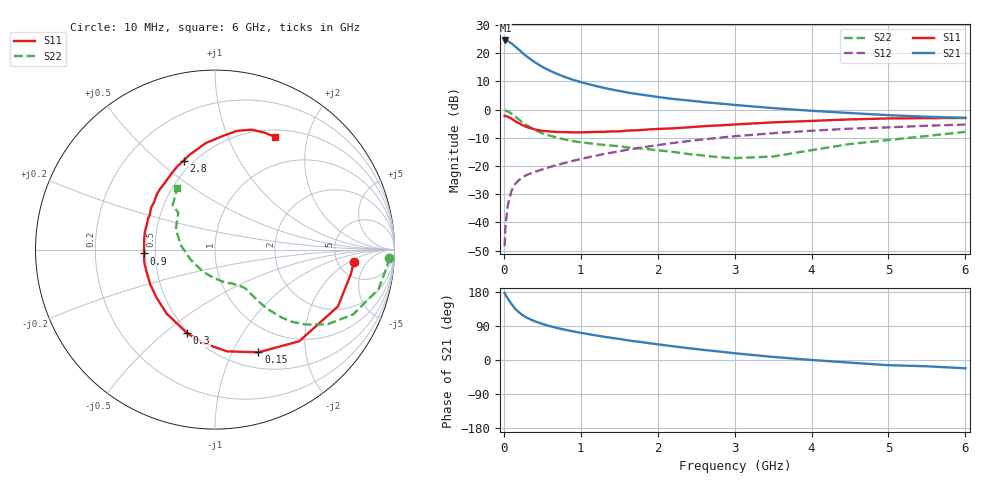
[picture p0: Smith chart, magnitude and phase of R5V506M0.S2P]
! SIEMENS Small Signal Semiconductors
! BFR183
! Si NPN RF Bipolar Junction Transistor in SOT23
! VCE = 0.5 V  IC = 6 mA
! Common Emitter S-Parameters:  May  1996
# GHz  S  MA  R  50
!  f  S11  S21  S12  S22
! GHz  MAG  ANG  MAG  ANG  MAG  ANG  MAG  ANG
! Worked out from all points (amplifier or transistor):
!   36 points, 10 MHz to 6 GHz, reference 50 ohm
!   highest |S21| = 24.5 dB at 20 MHz (marker M1)
!   |S21| within 3 dB of that: start of sweep to 184.2 MHz
!   unconditionally stable (mu >= 1): 830 MHz to 3.439 GHz
!   at 250 MHz: K = 0.49, MSG = 21.9 dB, |S12| = -23.9 dB
!   at 1.4 GHz: K = 1.10, MAG = 9.2 dB, |S12| = -15.2 dB
!   at 6 GHz: K = 0.98, MSG = 1.2 dB, |S12| = -5.3 dB
!   S11 on the Smith chart (normalised r, x): 10 MHz: 7.09, -2.47; 150 MHz: 0.68, -1.27; 300 MHz: 0.49, -0.60; 900 MHz: 0.43, -0.02; 2.8 GHz: 0.45, +0.61; 6 GHz: 0.59, +1.50
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0.01  0.7768 -5.1  16.82 176.8  0.0038 87.6  0.9727 -2.7
0.02  0.7691 -10.1  16.87 172.8  0.0082 86.9  0.9633 -5.5
0.05  0.7547 -24.8  16.56 162.7  0.0198 77.1  0.9375 -13.6
0.1  0.6935 -47.4  14.92 147.7  0.0365 66.9  0.8506 -25.1
0.15  0.6212 -67.1  13.12 134.6  0.0486 60.5  0.7522 -33.6
0.2  0.5708 -83.3  11.44 125.1  0.0571 55.9  0.6601 -39.3
0.25  0.5264 -96.3  9.904 117.6  0.064 52.8  0.5869 -43.2
0.3  0.4914 -108.3  8.724 111.4  0.0698 51.6  0.5286 -45.6
0.4  0.4467 -127.2  6.99 102.3  0.0788 50.5  0.4384 -48.6
0.5  0.4219 -140.4  5.735 95.2  0.0873 50.5  0.3801 -49.9
0.6  0.41 -151.5  4.899 89.3  0.0963 50.9  0.3456 -50.4
0.7  0.4015 -161.3  4.271 84.1  0.1052 51.7  0.3174 -51.0
0.9  0.3962 -176.9  3.383 75.5  0.1241 52.9  0.2764 -52.0
1.1  0.3996 170.6  2.834 68.3  0.1433 53.2  0.2548 -54.3
1.3  0.404 160.3  2.437 61.5  0.1635 52.6  0.2372 -56.7
1.6  0.4255 146.8  2.023 52.3  0.194 51.6  0.2155 -62.2
2.2  0.4665 126.4  1.549 36.2  0.2568 46.8  0.1784 -79.0
2.8  0.5254 109.4  1.286 22.4  0.3182 40.2  0.1434 -108.1
3.5  0.5954 95.0  1.066 8.1  0.3823 30.8  0.1477 -158.6
4.5  0.6724 79.6  0.871 -7.0  0.461 17.9  0.2458 152.5
5.5  0.7074 67.2  0.748 -16.6  0.5194 6.5  0.3416 133.6
6  0.7118 62.1  0.716 -21.9  0.5446 -1.0  0.404 121.4
